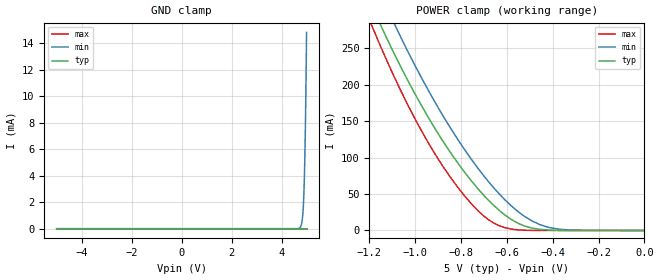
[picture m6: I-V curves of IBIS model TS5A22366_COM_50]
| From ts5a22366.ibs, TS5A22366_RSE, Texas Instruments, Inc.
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[Model]   TS5A22366_COM_50
Model_type  Terminator
| variable   typ   min   max
C_comp   120.97pF   78.63pF   148.45pF
| C_tri-state   120.97pF   78.63pF   148.45pF
[Temperature Range]   40   100   -40
| Ambient temperature   25   85   -40
[Voltage range]   5   4.5   5.5
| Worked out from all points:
|   POWER clamp passes 1 mA (typ) near -0.43 V on its own axis
[GND Clamp]
| TS5A22366_COM_50
|   Voltage   I(typ)   I(min)   I(max)
-5V       -16.55nA   -1.093uA   -6.1nA
4.725V    5.702nA    58.52uA    4.779nA
4.785V    5.782nA    254.1uA    4.843nA
4.83V     5.842nA    710.5uA    4.892nA
4.865V    5.891nA    1.51mA     4.93nA
4.895V    5.939nA    2.768mA    4.962nA
4.91V     5.968nA    3.68mA     4.978nA
4.925V    6.004nA    4.824mA    4.994nA
4.95V     6.098nA    7.325mA    5.021nA
4.975V    6.291nA    10.64mA    5.048nA
4.985V    6.426nA    12.2mA     5.059nA
5V        6.746nA    14.81mA    5.075nA
[POWER Clamp]
| TS5A22366_COM_50
|   Voltage   I(typ)   I(min)   I(max)
-5V       5.868A     5.842A     6.547A
-1.185V   305.9mA    349.2mA    278.2mA
-1.155V   285mA      327.8mA    255.8mA
-1.125V   264.7mA    306.9mA    234.2mA
-1.095V   245.1mA    286.6mA    213.4mA
-1.065V   226.1mA    266.9mA    193.4mA
-880mV    123.2mA    158.2mA    88.6mA
-755mV    68.2mA     97.84mA    36.69mA
-660mV    35.25mA    59.62mA    10.76mA
-550mV    9.67mA     25.63mA    810.5uA
-415mV    554.5uA    4.034mA    7.767uA
0V        0A         0A         0A
